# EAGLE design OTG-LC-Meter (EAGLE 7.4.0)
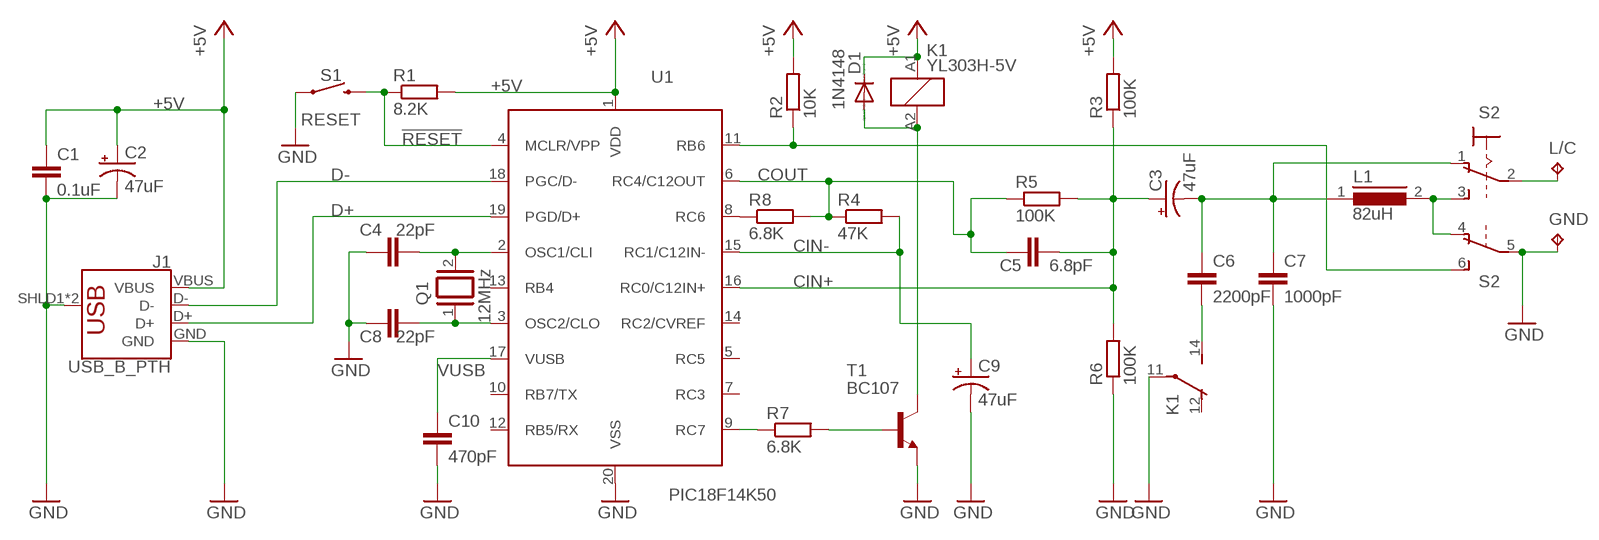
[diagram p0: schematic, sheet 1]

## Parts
C1  0.1uF  C-EU075-032X103  [C075-032X103]
C2  47uF  CPOL-USE5-6  [E5-6]
C3  47uF  CPOL-USE5-6  [E5-6]
C4  22pF  C-EU050-024X044  [C050-024X044]
C5  6.8pF  C-EU075-032X103  [C075-032X103]
C6  2200pF  C-EU150-054X183  [C150-054X183]
C7  1000pF  C-EU150-054X183  [C150-054X183]
C8  22pF  C-EU050-024X044  [C050-024X044]
C9  47uF  CPOL-USE5-6  [E5-6]
C10  470pF  C-EU075-032X103  [C075-032X103]
D1  1N4148  1N4148DO35-7  [DO35-7]
GND  TPPAD1-20  [P1-20]
J1  USB_B_PTH  [USB-B-PTH]
K1  YL303H-5V  ZNS5106  [ZN5]
L1  82uH  B82131  [SUKW1-17]
L/C  TPPAD1-20  [P1-20]
Q1  12MHz  XTAL/S  [QS]
R1  8.2K  R-EU_0207/10  [0207/10]
R2  10K  R-EU_0207/10  [0207/10]
R3  100K  R-EU_0207/10  [0207/10]
R4  47K  R-EU_0207/10  [0207/10]
R5  100K  R-EU_0207/10  [0207/10]
R6  100K  R-EU_0207/10  [0207/10]
R7  6.8K  R-EU_0207/10  [0207/10]
R8  6.8K  R-EU_M0805  [M0805]
S1  RESET  MOMENTARY-SWITCH-SPST-PTH-6.0MM  [TACTILE_SWITCH_PTH_6.0MM]
S2  M9040P2  [M9040P2]
T1  BC107  [TO18]
U1  PIC18F14K50  [DIL20]

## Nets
!RESET: R1.1 S1.3 U1.4(MCLR/VPP)
+5V: C1.1 C2.+ D1.C J1.VBUS K1.A1 R1.2 R2.2 R3.2 U1.1(VDD)
CIN+: C3.+ C5.2 R3.1 R5.2 R6.2 U1.16(RC0/C12IN+)
CIN-: C9.+ R4.2 U1.15(RC1/C12IN-)
COUT: C5.1 R4.1 R5.1 R8.2 U1.6(RC4/C12OUT)
D+: J1.D+ U1.19(PGD/D+)
D-: J1.D- U1.18(PGC/D-)
GND: C1.2 C2.- C4.1 C7.2 C8.1 C9.- C10.2 GND.TP J1.GND J1.SHLD1(SHIELD) J1.SHLD2(SHIELD) K1.11(2:P) R6.1 S1.1 S2.5(2:P) T1.1(E) U1.20(VSS)
N$1: R8.1 U1.8(RC6)
N$3: C4.2 Q1.2 U1.2(OSC1/CLI)
N$4: C8.2 Q1.1 U1.3(OSC2/CLO)
N$6: D1.A K1.A2 T1.3(C)
N$10: R7.2 T1.2(B)
N$11: R7.1 U1.9(RC7)
N$13: C6.2 K1.14(2:S)
N$14: C3.- C6.1 C7.1 L1.1 S2.1(1:O)
N$15: L1.2 S2.3(1:S) S2.4(2:O)
N$16: L/C.TP S2.2(1:P)
N$17: R2.1 S2.6(2:S) U1.11(RB6)
VUSB: C10.1 U1.17(VUSB)
Unconnected: K1.12(2:O) U1.5(RC5) U1.7(RC3) U1.10(RB7/TX) U1.12(RB5/RX) U1.13(RB4) U1.14(RC2/CVREF)

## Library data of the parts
C1 C4-C8 C10 = rcl:C-EU: CAPACITOR, European symbol
C2 C3 C9 = rcl:CPOL-US: POLARIZED CAPACITOR, American symbol
D1 = diode:1N4148: DIODE
GND L/C = testpad:TP: Test pad
J1 = SparkFun-Connectors:USB_B: USB Type B Connector SparkFun Products: SparkFun Stepoko PTH; PROD_ID: CONN-08278; SF_ID: PRT-00139
K1 = relay:ZNS5*: Miniature Power PCB Relay SCHRACK 1pole 10 A Source: http://www.schrack.com/.. 5847.pdf; OC_FARNELL: unknown; OC_NEWARK: unknown
L1 = inductors:B82131: INDUCTOR
Q1 = special:XTAL/S: CRYSTAL
R1-R8 = rcl:R-EU_: RESISTOR, European symbol
S1 = SparkFun-Switches:MOMENTARY-SWITCH-SPST: Momentary Switch (Pushbutton) - SPST; PROD_ID: SWCH-08441; SF_SKU: COM-00097
S2 = switch:M9040P2: TOGGLE SWITCH Marquardt
T1 = transistor:BC107: NPN TRANSISTOR
U1 = microchip:PIC18F14K50: 20-PIN Flash Microcontroller with XLP Technology

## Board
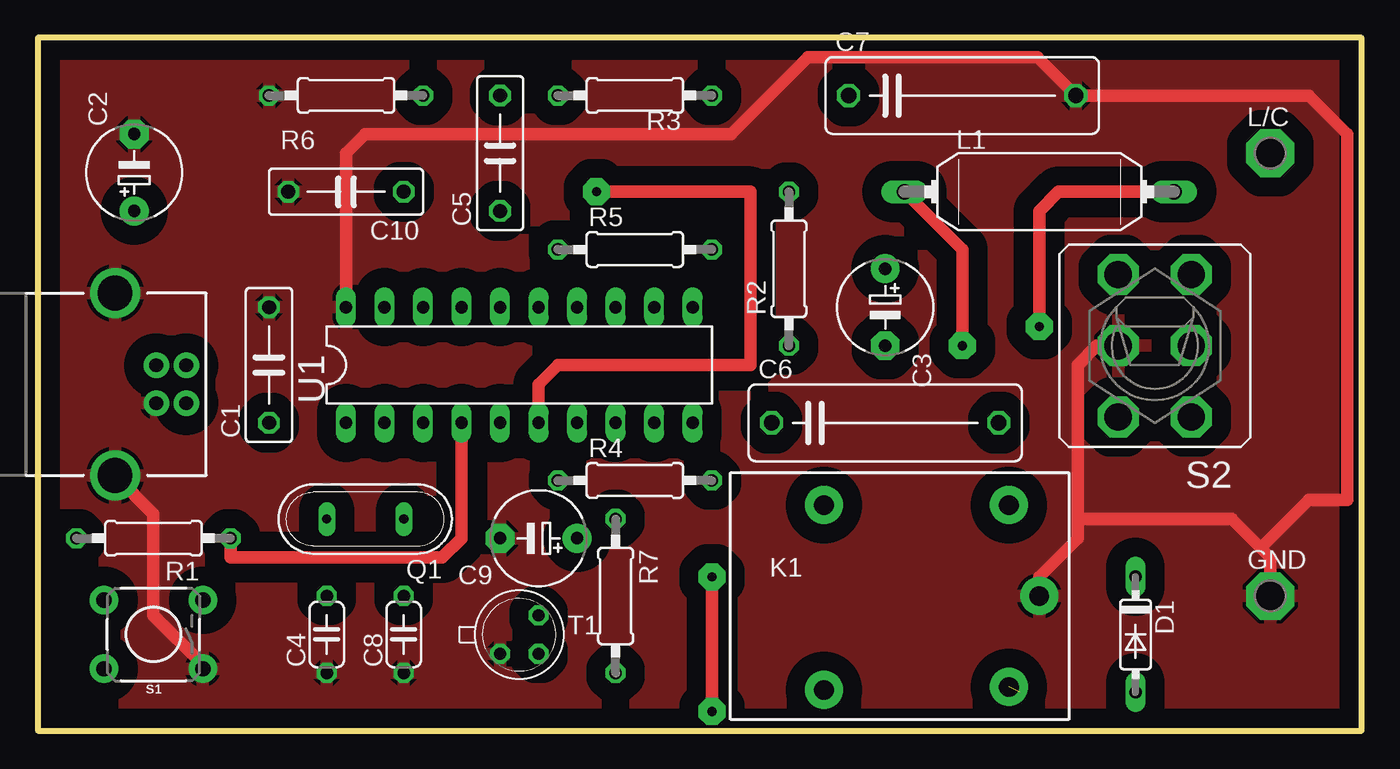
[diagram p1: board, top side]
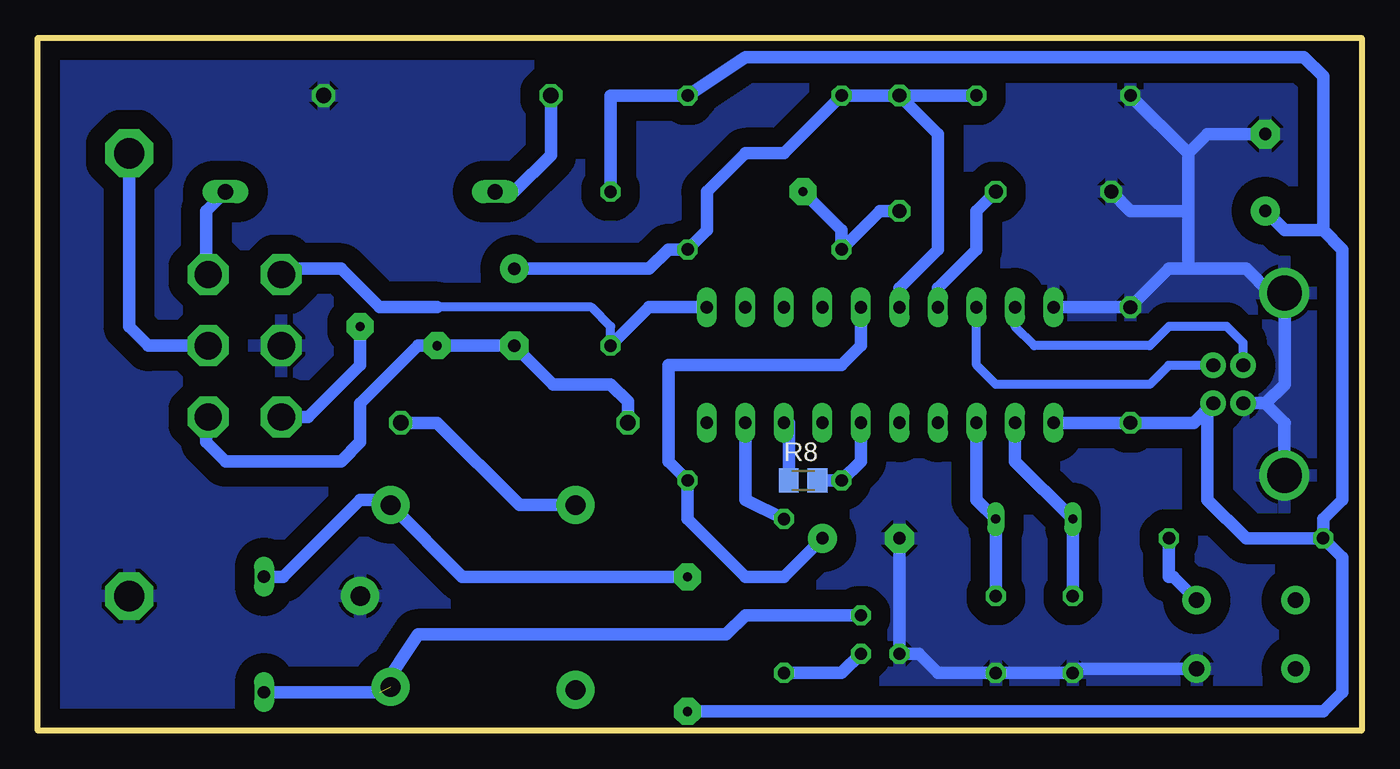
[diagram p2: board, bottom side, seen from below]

Size 87.3 x 45.71 mm. Coordinates in mm from the lower left corner, seen from the top.
Outline: 0,0 87.3,0 87.3,45.71 0,45.71 0,0
Copper layers (1*16): Top 0.035mm / dielectric 1.5mm / Bottom 0.035mm
Design rules "default": minimum track width 10mil, minimum drill 24mil, track to track 8mil, track to pad 8mil, pad to pad 8mil, via to via 8mil, smd to smd 8mil, copper to edge 40mil, drill to drill 8mil, minimum pad ring 10mil, minimum via ring 8mil, stop-mask expansion 4mil, vias tented up to drill 0mil, thermal gap 10mil

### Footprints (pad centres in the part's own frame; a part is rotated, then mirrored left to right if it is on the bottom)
C075-032X103 = drill 0.914 octagon: 1 -3.81,0; 2 3.81,0
E5-6 = drill 0.813 pad 1.905: + -2.54,0 | drill 0.813 pad 1.905 octagon: - 2.54,0
C050-024X044 = drill 0.813 octagon: 1 -2.54,0; 2 2.54,0
C150-054X183 = drill 1.016 octagon: 1 -7.493,0; 2 7.493,0
DO35-7 = drill 0.813 long: A 3.81,0; C -3.81,0
P1-20 = drill 2.007 pad 3.15 octagon: TP 0,0
USB-B-PTH = drill 0.914 pad 1.676: D+ 4,1.25; D- 5.981,1.25; GND 4,-1.25; VBUS 5.981,-1.25 | drill 2.286: SHLD1 1.282,-6.02; SHLD2 1.282,6.02
ZN5 = drill 1.3 pad 2.5: 11 8.89,0; 12 -5.31,-6.2; 14 -5.31,6; A1 6.89,6; A2 6.89,-6
SUKW1-17 = drill 1.016 long: 1 -8.89,0; 2 8.89,0
QS = drill 0.61 long: 1 -2.54,0; 2 2.54,0
0207/10 = drill 0.813 octagon: 1 -5.08,0; 2 5.08,0
M0805 = smd 1.3 x 1.6: 1 -0.95,0; 2 0.95,0
TACTILE_SWITCH_PTH_6.0MM = drill 1.016 pad 1.88: 1 -3.251,2.261; 2 3.251,2.261; 3 -3.251,-2.261; 4 3.251,-2.261
M9040P2 = drill 1.803 octagon: 1 -2.413,4.699; 2 -2.413,0; 3 -2.413,-4.699; 4 2.413,4.699; 5 2.413,0; 6 2.413,-4.699
TO18 = drill 0.813 octagon: 1 -1.27,-1.27; 2 1.27,-1.27; 3 1.27,1.27
DIL20 = drill 0.813 long: 1 -13.97,-3.81; 2 -11.43,-3.81; 3 -8.89,-3.81; 4 -6.35,-3.81; 5 -3.81,-3.81; 6 -1.27,-3.81; 7 1.27,-3.81; 8 3.81,-3.81; 9 6.35,-3.81; 10 8.89,-3.81; 11 8.89,3.81; 12 6.35,3.81; 13 3.81,3.81; 14 1.27,3.81; 15 -1.27,3.81; 16 -3.81,3.81; 17 -6.35,3.81; 18 -8.89,3.81; 19 -11.43,3.81; 20 -13.97,3.81

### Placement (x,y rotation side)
C1  15.24,24.13 90 top
C2  6.35,36.83 90 top
C3  55.88,27.94 270 top
C4  19.05,6.35 90 top
C5  30.48,38.1 90 top
C6  55.88,20.32 0 top
C7  60.96,41.91 0 top
C8  24.13,6.35 90 top
C9  33.02,12.7 180 top
C10  20.32,35.56 180 top
D1  72.39,6.35 270 top
GND  81.28,8.89 0 top
J1  3.81,22.86 0 top
K1  57.15,8.89 0 top
L1  66.04,35.56 0 top
L/C  81.28,38.1 0 top
Q1  21.59,13.97 180 top
R1  7.62,12.7 180 top
R2  49.53,30.48 90 top
R3  39.37,41.91 0 top
R4  39.37,16.51 0 top
R5  39.37,31.75 0 top
R6  20.32,41.91 0 top
R7  38.1,8.89 270 top
R8  36.83,16.51 0 bottom
S1  7.62,6.35 180 top
S2  73.66,25.4 180 top
T1  31.75,6.35 0 top
U1  34.29,24.13 0 top

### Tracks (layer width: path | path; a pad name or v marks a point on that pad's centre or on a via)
!RESET
  Top 0.813: U1.4 27.94,12.7 26.67,11.43 12.7,11.43 R1.1
  Bottom 0.813: S1.3 12.42,10.16 12.7,10.16 R1.1
+5V  (via drill 0.6 pad 1.78)
  Top 0.813: v44.45,10.16 v44.45,1.27
  Bottom 0.813: U1.1 C1.1 11.08,20.32 J1.VBUS 10.16,21.24 10.16,15.24 7.62,12.7 R1.2 | C2.+ 5.08,33.02 2.54,33.02 | 2.54,33.02 1.27,31.75 1.27,15.24 2.54,13.97 R1.2 | 2.54,33.02 2.54,43.18 3.81,44.45 40.64,44.45 R3.2 49.53,41.91 R2.2 | v44.45,10.16 59.31,10.16 K1.A1 64.39,15.24 66.04,15.24 71.12,10.16 D1.C | v44.45,1.27 2.54,1.27 1.27,2.54 1.27,11.43 R1.2
CIN+
  Bottom 0.813: C5.2 R3.1 38.1,38.1 40.64,38.1 43.18,35.56 43.18,33.02 R5.2 45.72,31.75 46.99,30.48 C3.+ | C5.2 R6.2 | C5.2 27.94,39.37 27.94,31.75 30.48,29.21 U1.16
CIN-
  Bottom 0.813: C9.+ 38.1,10.16 40.64,10.16 44.45,13.97 R4.2 45.72,17.78 45.72,24.13 34.29,24.13 33.02,25.4 U1.15
COUT  (via drill 0.6 pad 1.78)
  Top 0.813: U1.6 33.02,22.86 34.29,24.13 46.99,24.13 46.99,35.56 v36.83,35.56
  Bottom 0.813: U1.6 33.02,17.78 R4.1 R8.2 | v36.83,35.56 34.29,33.02 R5.1 31.75,34.29 C5.1
D+
  Bottom 0.61: J1.D+ 7.81,25.59 8.89,26.67 12.7,26.67 13.97,25.4 21.59,25.4 22.86,26.67 U1.19
D-
  Bottom 0.61: J1.D- 12.72,24.11 13.97,22.86 24.13,22.86 25.4,24.13 U1.18
GND
  Top 0.813: J1.SHLD1 7.62,14.31 7.62,7.62 10.87,4.37 S1.1 11.15,3.81 | U1.20 20.32,38.1 21.59,39.37 45.72,39.37 50.8,44.45 65.91,44.45 C7.2 83.82,41.91 86.36,39.37 86.36,15.24 83.82,15.24 80.64,12.06 | K1.11 66.04,10.16 68.58,12.7 68.58,13.97 | 68.58,13.97 68.58,24.13 69.85,25.4 S2.5 | GND.TP 81.28,11.43 80.64,12.06 | 80.64,12.06 78.74,13.97 68.58,13.97
  Bottom 0.813: J1.SHLD1 5.09,20.31 5.08,20.32 6.37,21.61 J1.GND 6.33,21.61 5.08,22.86 5.08,28.87 J1.SHLD2 6.02,28.88 7.62,30.48 11.43,30.48 | 11.43,30.48 12.7,30.48 C1.2 U1.20 | C2.- 10.16,39.37 11.43,38.1 | 11.43,38.1 11.43,34.29 | 11.43,34.29 11.43,30.48 | R6.1 11.43,38.1 | C10.2 15.24,34.29 11.43,34.29 | C9.- T1.1 29.21,5.08 27.94,3.81 C8.1 C4.1 18.77,4.09 S1.1
  pour Bottom (isolate 1.27): 0,0 87.63,0 87.63,45.72 0,45.72
  pour Top (isolate 1.27): 0,0 87.63,0 87.63,45.72 0,45.72
N$1
  Bottom 0.813: U1.8 37.78,20.32 R8.1
N$3
  Bottom 0.813: U1.2 22.86,17.78 Q1.2 C4.2
N$4
  Bottom 0.813: U1.3 25.4,15.24 Q1.1 C8.2
N$6  (1 unrouted)
  Bottom 0.813: T1.3 40.64,7.62 41.91,6.35 62.23,6.35 64.77,2.54 D1.A
N$10
  Bottom 0.813: T1.2 34.29,3.81 R7.2
N$11
  Bottom 0.813: U1.9 40.64,15.24 R7.1
N$13
  Bottom 0.813: K1.14 55.53,14.89 60.96,20.32 C6.2
N$14  (via drill 0.6 pad 1.78)
  Top 0.813: v60.96,25.4 60.96,31.75 L1.1
  Bottom 0.813: C7.1 53.47,37.97 55.88,35.56 L1.1 | C6.1 48.39,21.72 49.53,22.86 53.34,22.86 C3.- v60.96,25.4 62.23,25.4 66.04,21.59 66.04,19.05 67.31,17.78 74.93,17.78 76.2,19.05 76.2,20.57 S2.1
N$15  (via drill 0.6 pad 1.78)
  Top 0.813: v66.04,26.67 66.04,34.29 67.31,35.56 L1.2
  Bottom 0.813: S2.4 69.47,20.7 66.04,24.13 v66.04,26.67 | L1.2 76.2,34.29 76.2,30.23 S2.3
N$16
  Bottom 0.813: S2.2 80.01,25.4 81.28,26.67 L/C.TP
N$17
  Bottom 0.61: R2.1 49.53,26.67 50.8,27.94 60.96,27.94
  Bottom 0.813: U1.11 46.99,27.94 R2.1 | 60.96,27.94 64.77,27.94 67.31,30.48 70.87,30.48 S2.6
VUSB
  Bottom 0.813: C10.1 25.4,34.29 25.4,31.75 27.94,29.21 U1.17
